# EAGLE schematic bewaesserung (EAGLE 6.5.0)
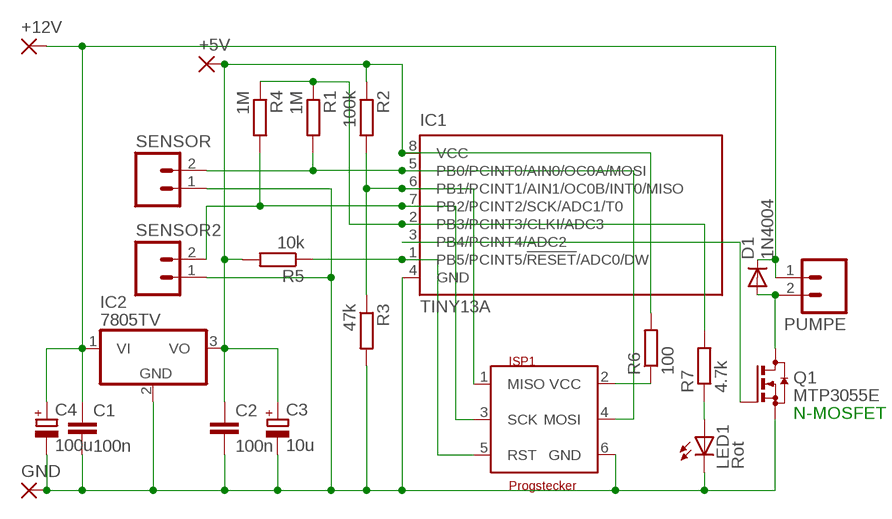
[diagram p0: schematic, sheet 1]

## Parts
+5V  2,54/1,0  [2,54/1,0]
+12V  2,54/1,0  [2,54/1,0]
C1  100n  C2,5-3  [C2.5-3]
C2  100n  C2,5-3  [C2.5-3]
C3  10u  CPOL-EUR/2012-12W  [R/2012-12W]
C4  100u  CPOL-EUE2.5-6  [E2,5-6]
D1  1N4004  [DO41-10]
GND  2,54/1,0  [2,54/1,0]
IC1  TINY13A  TINY13-20PU  [DIL08]
IC2  7805TV  [TO220V]
ISP1  Progstecker  ISP6N  [ISP6]
LED1  Rot  TLLG4400  [LED3MM]
PUMPE  M02  [02P]
Q1  MTP3055E  BSS123  [SOT23]
R1  1M  R-EU_M1206  [M1206]
R2  100k  R-EU_M1206  [M1206]
R3  47k  R-EU_M1206  [M1206]
R4  1M  R-EU_M1206  [M1206]
R5  10k  R-EU_M1206  [M1206]
R6  100  R-EU_R1206  [R1206]
R7  4.7k  R-EU_R0805  [R0805]
SENSOR  M02  [02P]
SENSOR2  M02  [02P]

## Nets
GND [dick2]: C1.2 C2.2 C3.- C4.- GND.1(P) IC1.4(GND) IC2.2(GND) ISP1.6(GND) LED1.K(C) Q1.2(S) R3.2 SENSOR2.1 SENSOR.1
N$2: +12V.1(P) C1.1 C4.+ D1.C IC2.1(VI) PUMPE.1
N$3: IC1.6(PB1/PCINT1/AIN1/OC0B/INT0/MISO) ISP1.1(MISO) R2.2 R3.1
N$4: IC1.5(PB0/PCINT0/AIN0/OC0A/MOSI) ISP1.4(MOSI) R1.2 SENSOR.2
N$5: IC1.3(PB4/PCINT4/ADC2) Q1.1(G)
N$6: D1.A PUMPE.2 Q1.3(D)
N$7: IC1.1(PB5/PCINT5/!RESET!/ADC0/DW) ISP1.5(RST) R5.1
N$8: IC1.2(PB3/PCINT3/CLKI/ADC3) R1.1 R4.1 R7.2
N$9: ISP1.2(VCC) R6.1
N$12: IC1.7(PB2/PCINT2/SCK/ADC1/T0) ISP1.3(SCK) R4.2 SENSOR2.2
N$15: LED1.A R7.1
VCC [dick]: +5V.1(P) C2.1 C3.+ IC1.8(VCC) IC2.3(VO) R2.1 R5.2 R6.2

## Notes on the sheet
- N-MOSFET

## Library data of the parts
+5V +12V GND = wirepad:2,54/1,0: THROUGH-HOLE PAD
C1 C2 = capacitor-wima:C: CAPACITOR
C3 C4 = rcl:CPOL-EU: POLARIZED CAPACITOR, European symbol
D1 = diode:1N4004: DIODE
IC1 = atmel:TINY13: 8-bit AVR Microcontroller with 1K Bytes In-System Programmable Flash Source: http://www.atmel.com/dyn/resources/prod_documents/2535S.pdf; MPN: ATTINY13-20PU; OC_FARNELL: 9171550; OC_NEWARK: 96K6521
IC2 = linear:78*: Positive VOLTAGE REGULATOR Source: http://cache.national.com/ds/LM/LM78L05.pdf http://www.fairchildsemi.com/ds/LM/LM7805.pdf
ISP1 = 6_stecker:ISP6: ISP-Stecker 6polig
LED1 = led:TLLG4400: Low Current (2mA) LED 3 mm Tinted Diffused Package color GREEN; MF: VISHAY SEMICONDUCTOR; OC_FARNELL: 1612435
PUMPE SENSOR SENSOR2 = con-amp-quick:M02: AMP QUICK CONNECTOR; OC_FARNELL: unknown; OC_NEWARK: unknown
Q1 = transistor-small-signal:BSS123: N-CHANNEL MOS FET
R1-R7 = rcl:R-EU_: RESISTOR, European symbol

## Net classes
1 dick: width 0.762 mm
2 dick2: width 1.016 mm, drill 0.762 mm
